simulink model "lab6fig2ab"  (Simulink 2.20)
settings: Solver=ode45  StartTime=0.0  StopTime=10.0  MaxStep=0.01  RelTol=1e-3  AbsTol=1e-6

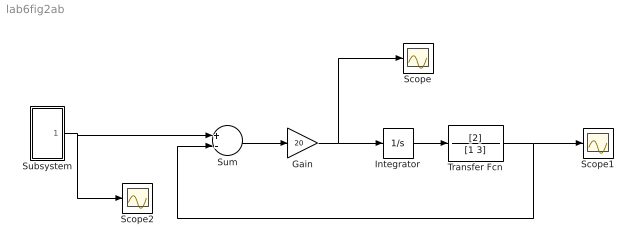
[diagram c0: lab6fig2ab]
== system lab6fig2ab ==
  Gain : Gain  Gain=20
  Integrator : Integrator  ExternalReset=none  InitialConditionSource=internal  InitialCondition=0  LimitOutput=off  UpperSaturationLimit=inf  LowerSaturationLimit=-inf  ShowSaturationPort=off  ShowStatePort=off  AbsoluteTolerance=auto
  Scope : Scope
  Scope1 : Scope
  Scope2 : Scope
  Subsystem : Subsystem
  Sum : Sum  Inputs=+-
  Transfer Fcn : TransferFcn  Numerator=[2]  Denominator=[1 3]
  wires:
  Sum/1 -> Gain/1
  Integrator/1 -> Transfer Fcn/1
  Gain/1 -> Integrator/1, Scope/1
  Transfer Fcn/1 -> Scope1/1, Sum/2
  Subsystem/1(Out1) -> Sum/1, Scope2/1

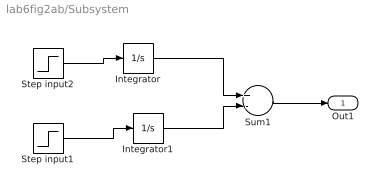
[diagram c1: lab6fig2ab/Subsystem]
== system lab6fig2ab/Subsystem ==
  Integrator : Integrator  ExternalReset=none  InitialConditionSource=internal  InitialCondition=0  LimitOutput=off  UpperSaturationLimit=inf  LowerSaturationLimit=-inf  ShowSaturationPort=off  ShowStatePort=off  AbsoluteTolerance=auto
  Integrator1 : Integrator  ExternalReset=none  InitialConditionSource=internal  InitialCondition=0  LimitOutput=off  UpperSaturationLimit=inf  LowerSaturationLimit=-inf  ShowSaturationPort=off  ShowStatePort=off  AbsoluteTolerance=auto
  Step input1 : Step  Time=1  Before=0  After=1
  Step input2 : Step  Time=0  Before=0  After=1
  Sum1 : Sum  Inputs=+-
  Out1 : Outport  Port=1
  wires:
  Sum1/1 -> Out1/1
  Step input2/1 -> Integrator/1
  Step input1/1 -> Integrator1/1
  Integrator/1 -> Sum1/1
  Integrator1/1 -> Sum1/2
